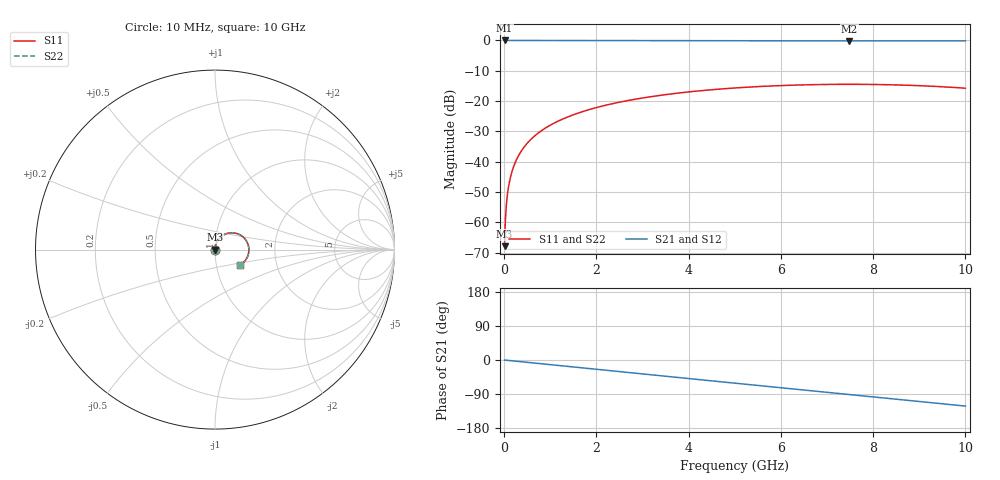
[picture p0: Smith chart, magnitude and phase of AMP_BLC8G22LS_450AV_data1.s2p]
! Created Fri Aug 16 14:40:27 2013
# ghz S ma R 50
! 2 Port Network Data from SP1.SP block
! freq  magS11  angS11  magS21  angS21  magS12  angS12  magS22  angS22
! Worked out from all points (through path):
!   1000 points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, 10 MHz to 10 GHz, reference 50 ohm
!   highest |S21| = 0.00 dB at 10 MHz (marker M1); lowest = -0.2 dB at 7.48 GHz (marker M2)
!   group delay of S21, straight-line fit = 33.7 ps
!   lowest |S11| = -67.9 dB at 10 MHz (marker M3), VSWR 1.00, Z = 50 + j0.0404 ohm
!   |S11| at or under -10 dB: start of sweep to end of sweep
!   |S22| runs from -67.9 to -14.5 dB; largest |S21 - S12| = 0
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0.01  0.0004035 89.9  1 -0.1  1 -0.1  0.0004035 89.9
0.03  0.00121 89.6  1 -0.4  1 -0.4  0.00121 89.6
0.07  0.002824 89.1  1 -0.9  1 -0.9  0.002824 89.1
0.08  0.003228 89.0  1 -1.0  1 -1.0  0.003228 89.0
0.1  0.004035 88.8  1 -1.2  1 -1.2  0.004035 88.8
0.13  0.005245 88.4  1 -1.6  1 -1.6  0.005245 88.4
0.17  0.006858 87.9  1 -2.1  1 -2.1  0.006858 87.9
0.23  0.009276 87.2  1 -2.8  1 -2.8  0.009276 87.2
0.37  0.01491 85.4  0.9999 -4.6  0.9999 -4.6  0.01491 85.4
0.58  0.02334 82.9  0.9997 -7.1  0.9997 -7.1  0.02334 82.9
0.87  0.03488 79.3  0.9994 -10.7  0.9994 -10.7  0.03488 79.3
1.23  0.049 74.9  0.9988 -15.1  0.9988 -15.1  0.049 74.9
1.68  0.06621 69.3  0.9978 -20.7  0.9978 -20.7  0.06621 69.3
2.42  0.09303 60.3  0.9957 -29.7  0.9957 -29.7  0.09303 60.3
3.34  0.123 49.0  0.9924 -41.0  0.9924 -41.0  0.123 49.0
5.01  0.1646 28.8  0.9864 -61.2  0.9864 -61.2  0.1646 28.8
5.84  0.1781 18.8  0.984 -71.2  0.984 -71.2  0.1781 18.8
6.67  0.1863 8.8  0.9825 -81.2  0.9825 -81.2  0.1863 8.8
7.48  0.189 -1.0  0.982 -91.0  0.982 -91.0  0.189 -1.0
8.34  0.1859 -11.4  0.9826 -101.4  0.9826 -101.4  0.1859 -11.4
9.14  0.1776 -21.1  0.9841 -111.1  0.9841 -111.1  0.1776 -21.1
10  0.1629 -31.6  0.9866 -121.6  0.9866 -121.6  0.1629 -31.6
